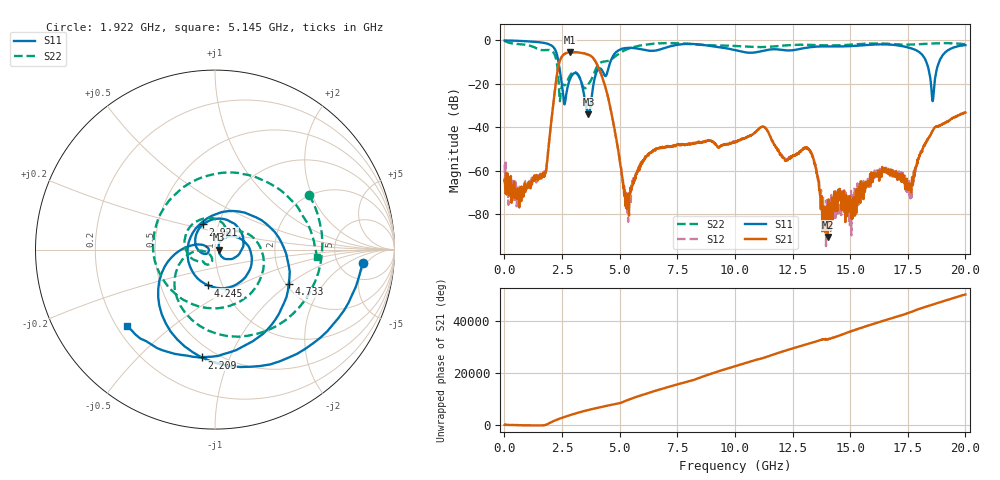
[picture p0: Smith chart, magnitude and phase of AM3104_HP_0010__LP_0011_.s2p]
!Created with skrf (http://scikit-rf.org).
# Hz S RI R 50.0
!freq ReS11 ImS11 ReS21 ImS21 ReS12 ImS12 ReS22 ImS22
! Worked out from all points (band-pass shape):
!   1601 points, 10 MHz to 20 GHz, reference 50 ohm
!   highest |S21| = -5.39 dB at 2.846 GHz (marker M1); lowest = -90.4 dB at 14.03 GHz (marker M2)
!   |S21| within 3 dB of the highest: 2.442 GHz to 3.871 GHz (1.429 GHz wide, 45.3 % of centre)
!   lowest |S11| = -33.9 dB at 3.646 GHz (marker M3), VSWR 1.04, Z = 52.1 + j0.037 ohm
!   |S11| at or under -10 dB: 2.35 GHz to 4.592 GHz (2.242 GHz wide, 64.6 % of centre); 18.31 GHz to 18.85 GHz (544.9 MHz wide, 2.93 % of centre)
!   |S22| runs from -27.9 to -0.2 dB; largest |S21 - S12| = 0.0038
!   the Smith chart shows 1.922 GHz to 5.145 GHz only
!   S11 on the Smith chart (normalised r, x): 1.922 GHz: 8.67, -4.00; 2.209 GHz: 0.42, -0.79; 2.921 GHz: 0.84, +0.24; 4.245 GHz: 0.86, -0.36; 4.733 GHz: 2.07, -1.00; 5.145 GHz: 0.24, -0.36
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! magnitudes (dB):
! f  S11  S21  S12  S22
! 10 MHz  0.0  -64.3  -57.0  -0.2
! 709.6 MHz  -0.2  -67.5  -69.0  -1.7
! 1.922 GHz  -1.7  -48.4  -48.2  -4.3
! 2.209 GHz  -4.4  -21.4  -21.4  -7.2
! 2.596 GHz  -29.1  -6.3  -6.3  -20.6
! 2.846 GHz  -17.8  -5.4  -5.4  -16.1
! 2.921 GHz  -16.2  -5.4  -5.4  -15.0
! 3.346 GHz  -19.5  -5.7  -5.7  -19.4
! 3.646 GHz  -33.9  -6.6  -6.6  -20.1
! 4.245 GHz  -13.8  -16.9  -16.9  -9.8
! 4.733 GHz  -6.9  -38.2  -38.2  -8.0
! 5.145 GHz  -3.7  -65.1  -64.8  -4.9
! 5.395 GHz  -3.4  -78.4  -74.3  -3.7
! 6.682 GHz  -4.3  -49.5  -49.6  -1.4
! 10.01 GHz  -4.4  -46.7  -46.4  -2.5
! 13.34 GHz  -3.0  -52.1  -52.7  -2.1
! 14.03 GHz  -2.7  -90.4  -80.1  -2.3
! 16.68 GHz  -1.8  -60.3  -59.3  -1.6
! 17.59 GHz  -3.4  -66.7  -67.6  -1.9
! 18.58 GHz  -27.9  -41.7  -41.7  -1.4
! 19.03 GHz  -6.6  -38.2  -38.3  -1.2
! 20 GHz  -2.2  -33.1  -33.0  -1.7
